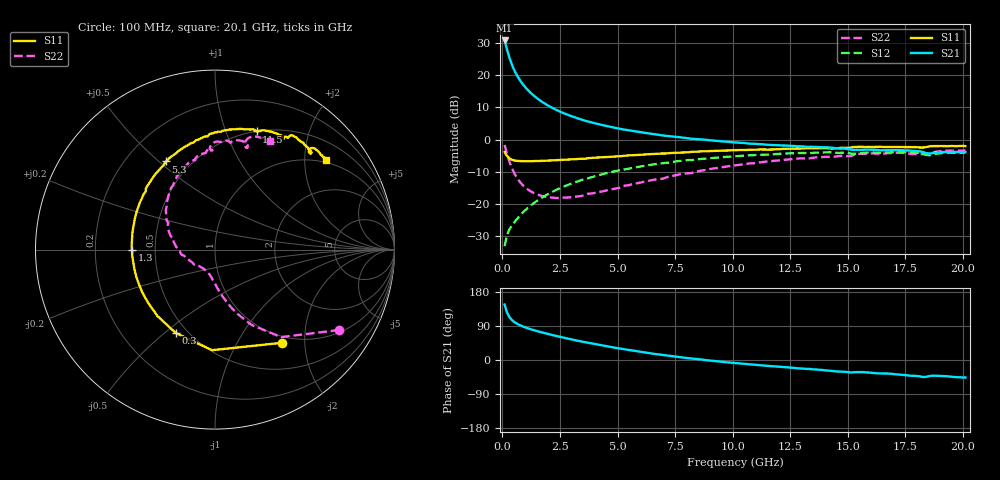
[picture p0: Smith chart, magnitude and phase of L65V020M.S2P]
!  Infineon Technologies AG
! BFR380L3 , PF131585-7, No.6, Th 09.10.01, soldered on pcb-board, measured with PP GSG850
!  Vce=5.0 V,  Ic=20.0 mA
! Common Emitter S-Parameters:  15. November 2001
#  GHz  S  MA  R  50
! f  S11  S21  S12  S22
! GHz  Mag  Ang  Mag  Ang  Mag  Ang  Mag  Ang
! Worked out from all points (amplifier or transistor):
!   201 points, 100 MHz to 20.1 GHz, reference 50 ohm
!   highest |S21| = 30.8 dB at 100 MHz (marker M1)
!   |S21| within 3 dB of that: start of sweep to 212.2 MHz
!   unconditionally stable (mu >= 1): 1.489 GHz to 4.356 GHz
!   at 3.4 GHz: K = 1.02, MAG = 8.6 dB, |S12| = -12.7 dB
!   at 10.1 GHz: K = 0.95, MSG = 2.1 dB, |S12| = -5.2 dB
!   at 20.1 GHz: K = 0.99, MSG = 0.1 dB, |S12| = -4.1 dB
!   S11 on the Smith chart (normalised r, x): 100 MHz: 0.89, -1.57; 300 MHz: 0.43, -0.55; 1.3 GHz: 0.37, -0.00; 5.3 GHz: 0.37, +0.53; 11.5 GHz: 0.50, +1.29; 20.1 GHz: 0.94, +2.52
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0.1  0.64 -54.2  34.64 146.4  0.02214 65.7  0.825 -32.9
0.2  0.5608 -91.8  25.38 125.8  0.03244 56.7  0.6109 -53.0
0.3  0.5134 -115.2  19.12 114.1  0.03993 54.3  0.465 -64.2
0.4  0.4898 -130.8  15.12 106.5  0.0456 54.3  0.372 -71.5
0.5  0.4759 -141.7  12.41 101.2  0.05091 55.7  0.3104 -76.5
0.6  0.47 -149.7  10.51 97.1  0.05659 57.1  0.2677 -80.5
0.7  0.4652 -156.3  9.112 93.7  0.06223 58.4  0.2362 -83.8
0.8  0.4636 -161.4  8.025 90.8  0.06829 59.7  0.2128 -86.7
0.9  0.462 -166.0  7.172 88.2  0.07424 60.6  0.1943 -89.2
1.1  0.4612 -173.4  5.926 83.8  0.0866 62.0  0.1694 -94.2
1.3  0.4623 -179.5  5.047 79.9  0.099 62.7  0.1524 -98.5
1.7  0.4669 170.8  3.907 73.0  0.1245 63.0  0.1339 -107.2
2.2  0.4764 161.0  3.064 65.4  0.1565 61.9  0.1255 -117.8
2.8  0.4894 151.0  2.459 57.1  0.1948 59.6  0.1259 -130.1
3.5  0.5035 140.5  2.009 48.1  0.2393 56.0  0.1351 -141.9
5.3  0.5615 119.0  1.431 28.4  0.3431 44.9  0.1923 -173.3
6.8  0.6037 103.7  1.184 14.4  0.4244 34.8  0.2443 164.9
10.1  0.6838 78.9  0.9025 -8.0  0.5513 13.3  0.3984 130.5
11.5  0.6979 70.6  0.831 -15.4  0.5842 4.3  0.4577 117.7
13.5  0.7305 61.2  0.7719 -24.7  0.6234 -7.6  0.5219 101.8
16.8  0.7698 48.8  0.6888 -35.9  0.6332 -23.9  0.6173 79.8
20.1  0.7925 38.9  0.6425 -46.1  0.6265 -37.9  0.6778 63.0
